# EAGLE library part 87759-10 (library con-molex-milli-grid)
HEADER
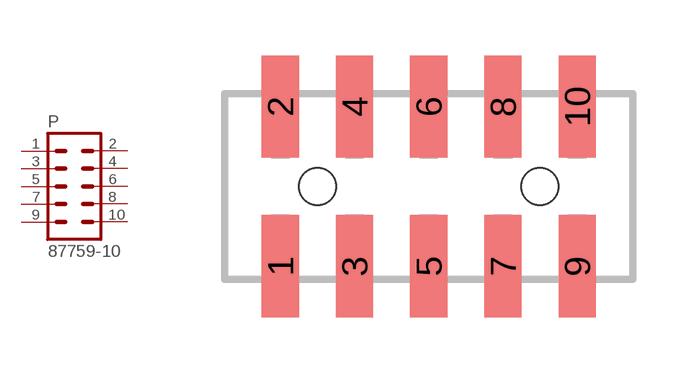
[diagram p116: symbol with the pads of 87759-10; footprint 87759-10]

Designator prefix P

## 87759-10  [87759-10]
1  1  pas
2  2  pas
3  3  pas
4  4  pas
5  5  pas
6  6  pas
7  7  pas
8  8  pas
9  9  pas
10  10  pas

## Footprint 87759-10 (pad centres in mm)
HEADER SMD Dual Row, Vertical
smd 1 x 2.75: 1 -4,-2.15; 2 -4,2.15; 3 -2,-2.15; 4 -2,2.15; 5 0,-2.15; 6 0,2.15; 7 2,-2.15; 8 2,2.15; 9 4,-2.15; 10 4,2.15
hole 1 at -3,0
hole 1 at 3,0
